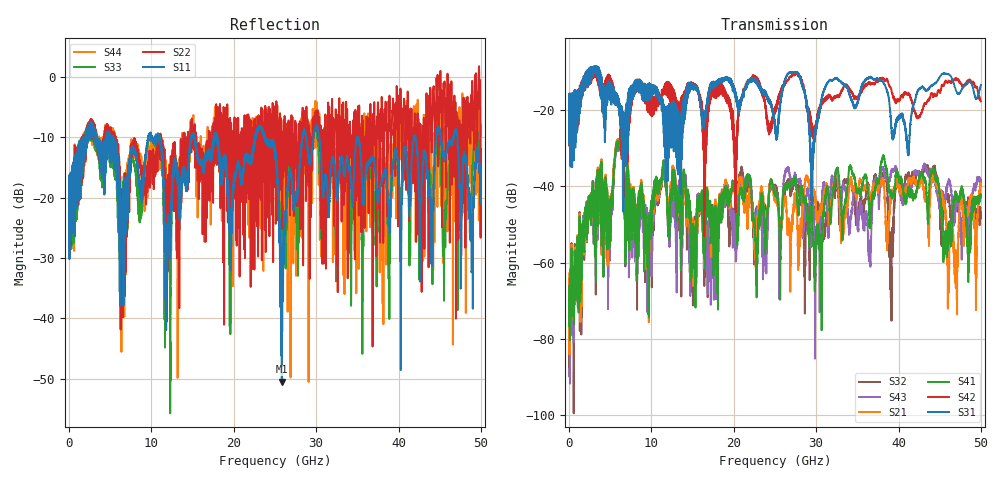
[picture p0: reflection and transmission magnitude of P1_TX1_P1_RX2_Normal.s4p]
!Keysight Technologies,N5225B,MY57041031,A.13.20.10
!Date: Friday, May 31, 2019 11:15:23
!Correction: S11(Full 4 Port(1,2,3,4))
!S12(Full 4 Port(1,2,3,4))
!S13(Full 4 Port(1,2,3,4))
!S14(Full 4 Port(1,2,3,4))
!S21(Full 4 Port(1,2,3,4))
!S22(Full 4 Port(1,2,3,4))
!S23(Full 4 Port(1,2,3,4))
!S24(Full 4 Port(1,2,3,4))
!S31(Full 4 Port(1,2,3,4))
!S32(Full 4 Port(1,2,3,4))
!S33(Full 4 Port(1,2,3,4))
!S34(Full 4 Port(1,2,3,4))
!S41(Full 4 Port(1,2,3,4))
!S42(Full 4 Port(1,2,3,4))
!S43(Full 4 Port(1,2,3,4))
!S44(Full 4 Port(1,2,3,4))
!S4P File: Measurements: <S11,S12,S13,S14>,
!<S21,S22,S23,S24>,
!<S31,S32,S33,S34>,
!<S41,S42,S43,S44>:
# Hz S  dB  R 50.0
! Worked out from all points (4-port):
!   5000 points, 10 MHz to 50 GHz, reference 50 ohm
!   strongest paths, dB at 10 MHz, 12.51 GHz, 25.01 GHz, 37.51 GHz, 50 GHz:
!     S31: -19.3, -29.2, -24.6, -11.8, -13.5
!     S42: -19.4, -16.4, -19.2, -12.5, -17.7
!     S41: -66.2, -38.8, -41.6, -39.0, -42.4
!     S21: -62.8, -36.8, -42.2, -41.1, -39.4
!     S43: -77.8, -39.8, -41.2, -41.4, -39.0
!     S32: -87.4, -38.5, -40.6, -41.5, -47.8
!   lowest |S11| = -50.5 dB at 25.83 GHz (marker M1), VSWR 1.01, Z = 50 + j0.3 ohm
!   |S11| at or under -10 dB: 18.01 GHz to 22.61 GHz (4.596 GHz wide, 22.6 % of centre); 30.38 GHz to 34.94 GHz (4.563 GHz wide, 14 % of centre); 34.98 GHz to 41.82 GHz (6.84 GHz wide, 17.8 % of centre)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
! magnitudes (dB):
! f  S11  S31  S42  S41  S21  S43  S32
! 10 MHz  -19.9  -19.3  -19.4  -66.2  -62.8  -77.8  -87.4
! 5.95 GHz  -17.1  -19.0  -18.1  -28.7  -28.3  -29.3  -28.8
! 9.46 GHz  -11.3  -17.5  -19.1  -52.8  -56.6  -47.3  -49.3
! 23.31 GHz  -8.3  -14.8  -14.6  -44.4  -42.8  -45.0  -45.4
! 25.83 GHz  -50.5  -16.0  -14.7  -47.9  -49.1  -48.9  -49.5
! 28.56 GHz  -8.6  -15.0  -14.6  -44.2  -41.4  -47.8  -59.1
! 50 GHz  -19.6  -13.5  -17.7  -42.4  -39.4  -39.0  -47.8
